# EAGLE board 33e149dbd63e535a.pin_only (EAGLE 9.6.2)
REV: D

Size 50.8 x 10.16 mm. Coordinates in mm from the lower left corner, seen from the top.
Outline: 0,0 50.8,0 50.8,10.16 0,10.16 0,0
Copper layers (1*16): Top 0.035mm / dielectric 1.5mm / Bottom 0.035mm
Design rules "adafruit *": minimum track width 8mil, minimum drill 15.5mil, track to track 8mil, track to pad 8mil, pad to pad 8mil, via to via 8mil, smd to smd 8mil, copper to edge 10mil, drill to drill 8mil, minimum pad ring 10mil, minimum via ring 8mil, stop-mask expansion 4mil, vias tented up to drill 20mil, thermal gap 10mil

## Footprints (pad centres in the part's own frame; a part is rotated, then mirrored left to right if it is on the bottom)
0603-NO = smd 1.075 x 1: 1 -0.85,0; 2 0.85,0
1X4-SMT = smd 1.27 x 2.54: 1 -3.81,0; 2 -1.27,0; 3 1.27,0; 4 3.81,0
FIDUCIAL_1MM = smd 1 x 1: 1 0,0
WS2812B-NARROW = smd 1.3 x 1.2: 1-VDD 2.35,-1.65; 2-DOUT 2.35,1.65; 3-GND -2.35,1.65; 4-DIN -2.35,-1.65
MOUNTINGHOLE_2.0_PLATED = drill 2.2 pad 3: P$1 0,0

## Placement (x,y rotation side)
C1  1.0uF  [0603-NO]  8.38,8.38 180 top
C2  1.0uF  [0603-NO]  16.89,8.38 180 top
C3  1.0uF  [0603-NO]  22.23,8.38 180 top
C4  1.0uF  [0603-NO]  28.57,8.38 180 top
C5  1.0uF  [0603-NO]  33.66,8.38 180 top
C6  1.0uF  [0603-NO]  42.04,8.38 180 top
C7  1.0uF  [0603-NO]  48.26,8.38 180 top
CN1  1X4SMT  [1X4-SMT]  49.4,5.08 270 bottom
CN2  1X4SMT  [1X4-SMT]  1.4,5.08 90 bottom
FID1  FIDUCIAL_1MM  [FIDUCIAL_1MM]  5.33,8.38 0 top
FID3  FIDUCIAL_1MM  [FIDUCIAL_1MM]  45.09,8.38 0 top
LED1  SKC6812  [WS2812B-NARROW]  3.17,3.81 0 top
LED2  SKC6812  [WS2812B-NARROW]  9.53,3.81 0 top
LED3  SKC6812  [WS2812B-NARROW]  15.88,3.81 0 top
LED4  SKC6812  [WS2812B-NARROW]  22.23,3.81 0 top
LED5  SKC6812  [WS2812B-NARROW]  28.57,3.81 0 top
LED6  SKC6812  [WS2812B-NARROW]  34.92,3.81 0 top
LED7  SKC6812  [WS2812B-NARROW]  41.27,3.81 0 top
LED8  SKC6812  [WS2812B-NARROW]  47.62,3.81 0 top
PLABEL0  [PLABEL0]  7.62,3.17 0 bottom
PLABEL1  [PLABEL1]  6.99,0.51 0 bottom
PLABEL2  [PLABEL2]  6.1,5.59 0 bottom
PLABEL3  [PLABEL3]  47.88,3.17 0 bottom
PLABEL4  [PLABEL4]  47.88,5.71 0 bottom
PLABEL5  [PLABEL5]  47.88,0.64 0 bottom
PLABEL6  [PLABEL6]  6.99,8.13 0 bottom
PLABEL7  [PLABEL7]  47.88,8.26 0 bottom
PLABEL8  [PLABEL8]  34.29,6.6 0 bottom
PLABEL9  [PLABEL9]  35.56,8.89 0 bottom
R1  470 ohm  [0603-NO]  2.41,8.38 0 top
U$1  [ADAFRUIT_TEXT_20MM]  39.37,0.13 0 bottom
U$2  MOUNTINGHOLE2.0  [MOUNTINGHOLE_2.0_PLATED]  12.7,8.13 0 top
U$3  MOUNTINGHOLE2.0  [MOUNTINGHOLE_2.0_PLATED]  38.1,8.13 0 top
U$4  [ADAFRUIT_2.5MM]  24.26,7.49 0 top
U$5  [PCBFEAT-REV-040]  18.41,1.91 0 bottom

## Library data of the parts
C1-C7 R1 U$1 U$4 = microbuilder
CN1 CN2 = adafruit
FID1 FID3 = microbuilder; BOM: EXCLUDE
LED1-LED8 U$5 = microbuilder; ROT: 180
PLABEL0 PLABEL1-PLABEL9 = pinguin
U$2 U$3 = adafruit_electromech; BOM: EXCLUDE

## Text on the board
Pinguin_bBackup: GND | Cool/Warm/Amber | GND | DIN | DOUT | 8 NeoPixel Stick | 5VDC | 5VDC | GND | GND

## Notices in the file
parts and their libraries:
microbuilder: This work is placed in the public domain, and may be freely used for commercial and non-commercial work with the following conditions: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
